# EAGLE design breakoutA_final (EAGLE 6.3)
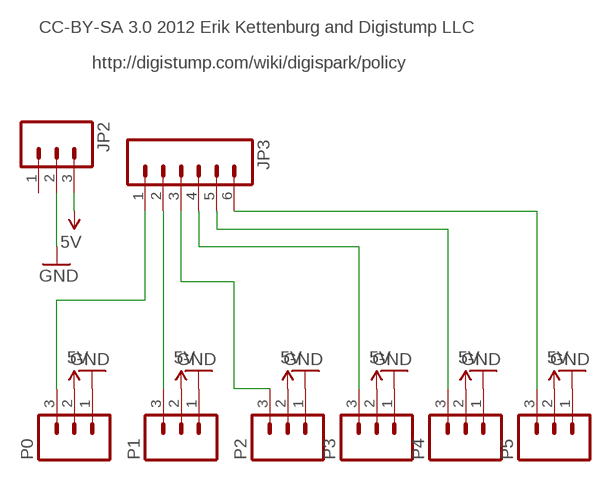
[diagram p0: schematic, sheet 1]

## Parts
JP2  M03PTH  [1X03]
JP3  M06SIP  [1X06]
P0  M03PTH  [1X03]
P1  M03PTH  [1X03]
P2  M03PTH  [1X03]
P3  M03PTH  [1X03]
P4  M03PTH  [1X03]
P5  M03PTH  [1X03]

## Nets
5V: JP2.3 P0.2 P1.2 P2.2 P3.2 P4.2 P5.2
GND: JP2.2 P0.1 P1.1 P2.1 P3.1 P4.1 P5.1
N$1: JP3.1 P0.3
N$2: JP3.2 P1.3
N$3: JP3.3 P2.3
N$4: JP3.4 P3.3
N$5: JP3.5 P4.3
N$6: JP3.6 P5.3
Unconnected: JP2.1

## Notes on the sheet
- CC-BY-SA 3.0 2012 Erik Kettenburg and Digistump LLC
- http://digistump.com/wiki/digispark/policy

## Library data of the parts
JP2 P0 P1-P5 = SparkFun:M03: Header 3 Standard 3-pin 0.1" header. Use with straight break away headers (SKU : PRT-00116), right angle break away headers (PRT-00553), swiss pins (PRT-00743), machine pins (PRT-00117), and female headers (PRT-00115). Molex polarized connector foot print use with SKU : PRT-08232 with associated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
JP3 = SparkFun:M06: Header 6 Standard 6-pin 0.1" header. Use with straight break away headers (SKU : PRT-00116), right angle break away headers (PRT-00553), swiss pins (PRT-00743), machine pins (PRT-00117), and female headers (PRT-00115). Molex polarized connector foot print use with SKU : PRT-08094 with associated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

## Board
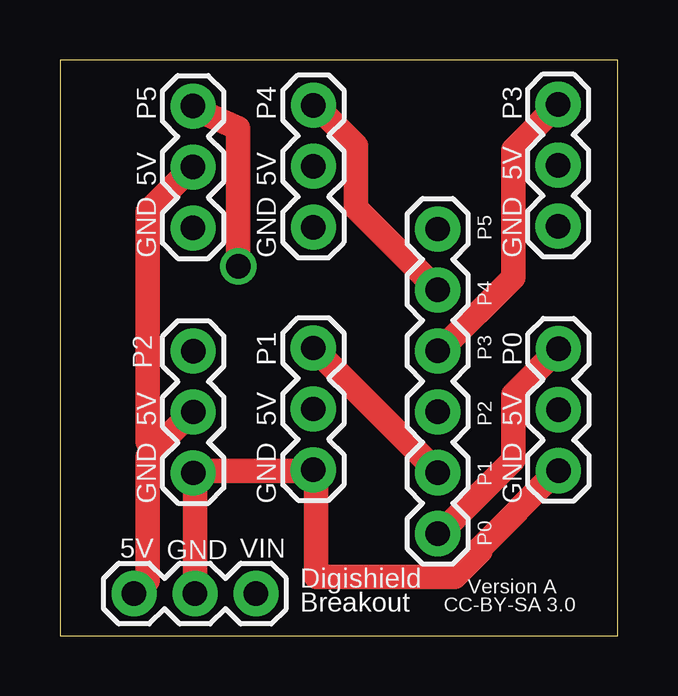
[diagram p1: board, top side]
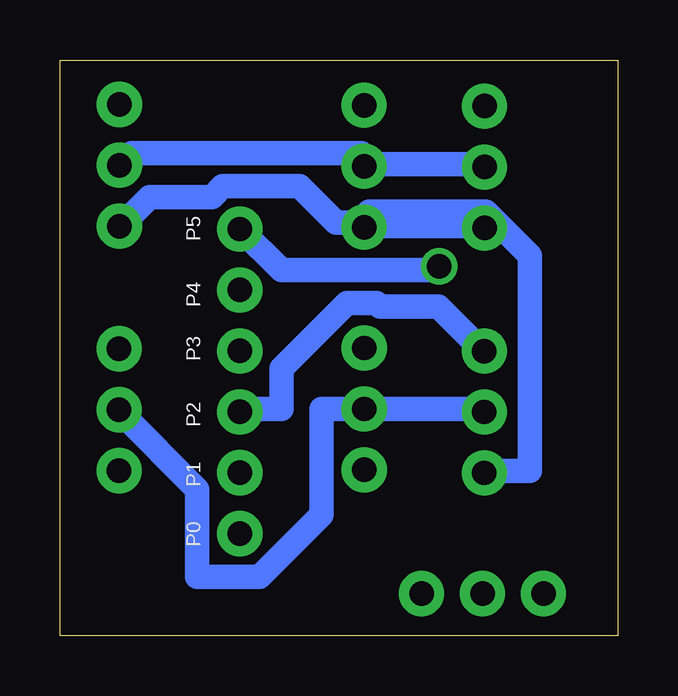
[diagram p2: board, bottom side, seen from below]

Size 23.25 x 24 mm. Coordinates in mm from the lower left corner, seen from the top.
Outline: 0,24 0,0 23.25,0 23.25,24 0,24
Copper layers (1*16): Top 0.0356mm / dielectric 1.5011mm / Bottom 0.0356mm
Design rules "default": minimum track width 40mil, minimum drill 40mil, track to track 12mil, track to pad 12mil, pad to pad 12mil, via to via 12mil, smd to smd 8mil, copper to edge 15mil, drill to drill 12mil, minimum pad ring 7mil, minimum via ring 7mil, stop-mask expansion 4mil, vias tented up to drill 25mil, thermal gap 10mil

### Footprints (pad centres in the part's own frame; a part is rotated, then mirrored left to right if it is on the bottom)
1X03 = drill 1.016 pad 1.88: 1 0,0; 2 2.54,0; 3 5.08,0
1X06 = drill 1.016 pad 1.88: 1 0,0; 2 2.54,0; 3 5.08,0; 4 7.62,0; 5 10.16,0; 6 12.7,0

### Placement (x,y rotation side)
JP2  8.17,1.75 180 top
JP3  15.75,4.25 90 top
P0  20.79,6.88 90 top
P1  10.56,6.91 90 top
P2  5.56,6.78 90 top
P3  20.77,17.07 90 top
P4  10.57,17.03 90 top
P5  5.55,17 90 top

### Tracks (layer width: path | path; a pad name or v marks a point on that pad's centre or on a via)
5V
  Top 1.016: 3.96,7.77 5.49,9.3 P2.2 | 3.96,7.77 3.66,7.47 3.66,2.29 3.2,1.83 JP2.3 | P5.2 5.49,19.51 3.66,17.68 3.66,8.08 3.96,7.77
  Bottom 1.016: P5.2 5.64,19.66 10.52,19.66 P4.2 10.67,20.12 20.27,20.12 20.73,19.66 P3.2 | P0.2 20.73,9.3 17.53,6.1 17.53,2.44 14.94,2.44 12.34,5.03 12.34,9.45 10.67,9.45 P1.2 10.06,9.45 5.64,9.45 P2.2
GND
  Top 1.016: JP2.2 5.64,1.83 5.64,6.4 P2.1 5.64,6.86 10.52,6.86 P1.1 10.67,6.4 10.67,2.44 16.46,2.44 17.53,3.5 17.53,3.66 20.73,6.86 P0.1
  Bottom 1.016: P5.1 5.64,17.07 10.52,17.07 P4.1 | P3.1 20.73,17.07 19.51,18.29 16.92,18.29 16.46,18.75 13.26,18.75 11.73,17.22 10.97,17.22 P4.1 | P4.1 10.52,17.53 10.36,17.68 5.49,17.68 3.66,15.85 3.66,6.86 5.49,6.86 P2.1
N$1
  Top 1.016: JP3.1 15.85,4.27 18.9,7.32 18.9,10.06 20.73,11.89 P0.3
N$2
  Top 1.016: JP3.2 15.7,6.86 10.67,11.89 P1.3
N$3
  Bottom 1.016: P2.3 5.64,11.89 7.47,13.72 9.91,13.72 10.06,13.87 11.28,13.87 14.02,11.12 14.02,9.45 15.7,9.45 JP3.3
N$4
  Top 1.016: JP3.4 15.85,11.89 18.9,14.94 18.9,20.27 20.73,22.1 P3.3
N$5
  Top 1.016: JP3.5 15.7,14.48 12.34,17.83 12.34,20.42 10.67,22.1 P4.3
N$6  (via drill 1.02)
  Top 1.016: v7.44,15.39 7.44,21.15 5.64,21.95 P5.3
  Bottom 1.016: v7.44,15.39 7.59,15.24 14.02,15.24 15.7,16.92 JP3.6

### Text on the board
tPlace: Digishield | Version A | CC-BY-SA 3.0
tNames: P5 | P4 | P3 | 5V | 5V | 5V | GND | GND | P5 | GND | P4 | P3 | P2 | P1 | P0 | 5V | 5V | P2 | 5V | GND | GND | P1 | GND | GND | P0 | 5V | VIN | Breakout
bNames: P5 | P4 | P3 | P2 | P1 | P0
